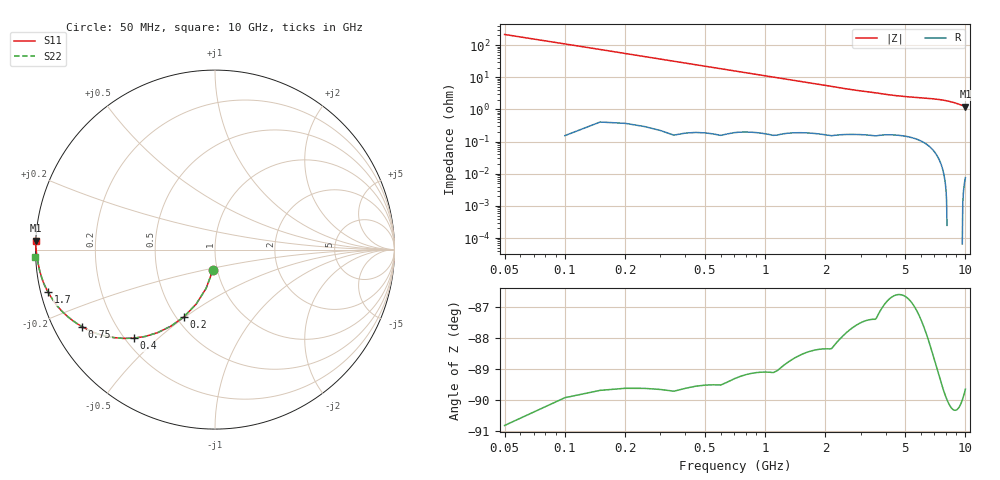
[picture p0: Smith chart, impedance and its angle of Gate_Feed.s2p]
! Created Fri Sep 21 12:41:52 2018
# ghz S ma R 50
! 2 Port Network Data from SP1.SP block
! freq  magS11  angS11  magS21  angS21  magS12  angS12  magS22  angS22
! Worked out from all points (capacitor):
!   200 points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, 50 MHz to 10 GHz, reference 50 ohm
!   read as one part in shunt: C = 14.4 pF near 100 MHz
!   lowest |Z| = 1.21 ohm at 10 GHz (marker M1)
!   S11 on the Smith chart (normalised r, x): 50 MHz: 0.95, -0.22; 200 MHz: 0.55, -0.49; 400 MHz: 0.23, -0.42; 750 MHz: 0.08, -0.27; 1.7 GHz: 0.02, -0.12; 10 GHz: -0.00, +0.02
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0.05  0.1154 -95.9  0.9949 -6.6  0.9949 -6.6  0.1154 -95.6
0.1  0.2219 -102.9  0.9746 -12.9  0.9746 -12.9  0.2219 -102.9
0.15  0.3213 -109.1  0.9451 -18.8  0.9451 -18.8  0.3213 -109.1
0.2  0.4114 -114.7  0.9085 -24.4  0.9085 -24.4  0.4115 -114.8
0.25  0.4914 -119.9  0.8675 -29.5  0.8675 -29.5  0.4915 -119.9
0.3  0.5612 -124.6  0.8241 -34.2  0.8241 -34.2  0.5612 -124.6
0.4  0.6701 -132.6  0.7376 -42.2  0.7376 -42.2  0.6701 -132.6
0.55  0.777 -141.7  0.6225 -51.2  0.6225 -51.2  0.777 -141.7
0.65  0.8234 -146.2  0.5586 -55.6  0.5586 -55.6  0.8235 -146.2
0.75  0.8561 -149.9  0.505 -59.1  0.505 -59.1  0.8561 -149.9
0.95  0.9005 -155.4  0.4202 -64.5  0.4202 -64.5  0.9006 -155.5
1.15  0.9279 -159.4  0.357 -68.5  0.357 -68.5  0.9279 -159.4
1.7  0.9601 -165.8  0.2529 -74.3  0.2529 -74.3  0.9602 -165.9
1.75  0.9618 -166.2  0.2464 -74.6  0.2464 -74.6  0.962 -166.3
2.55  0.9782 -170.9  0.1711 -78.7  0.1711 -78.7  0.9785 -170.9
3.4  0.9842 -173.3  0.1348 -80.7  0.1348 -80.7  0.9844 -173.3
4.2  0.9866 -174.9  0.1119 -81.6  0.1119 -81.6  0.9869 -174.9
5.05  0.9885 -176.0  0.09915 -82.6  0.09915 -82.6  0.9886 -175.8
6.7  0.9932 -178.1  0.08665 -85.7  0.08665 -85.7  0.9924 -176.6
8.35  0.9972 179.3  0.07081 -89.1  0.07081 -89.1  0.9979 -177.1
9.15  0.9987 178.1  0.06022 -89.9  0.06022 -89.9  1 -177.3
10  1 177.2  0.04865 -89.9  0.04865 -89.9  1.002 -177.7
